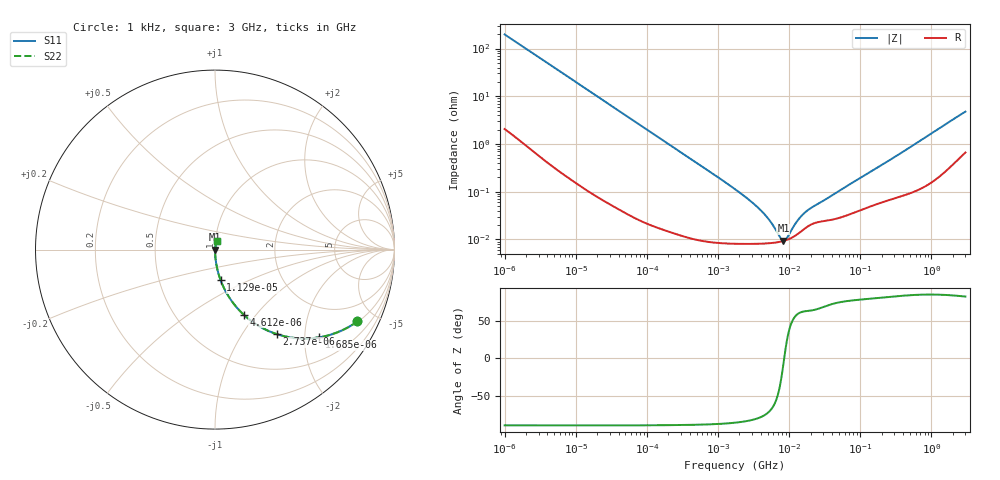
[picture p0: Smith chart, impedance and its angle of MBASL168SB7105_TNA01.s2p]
! MBASL168SB7105_TNA01  S-PARAMETER MODEL  ( Standard Model )
! Model Generated by TAIYO YUDEN Corporation (http://www.ty-top.com)
! Version 1.0
! TAIYO YUDEN Control No. 220601
! Copyright(c) 2012 TAIYO YUDEN CO.,LTD. All Rights Reserved.
! Product Description (link to TY-COMPAS)
! https://ds.yuden.co.jp/TYCOMPAS/or/detail?pn=MBASL168SB7105KTNA01&u=M
! Products Name : Multilayer Ceramic Capacitors
! Characteristics :
!  Capacitance : 1 [uF] , Rated Voltage : 10 [V] , TCC : X7R
!  Case Size : 1.6 x 0.8 / 0.063 x 0.031 [mm/inch] , Thickness : 0.8 / 0.031 [mm/inch]
!  (Conditions: Temperature = 25 [degC] , DC Bias Voltage = 0 [V])
! External Node Assignments :
!  1  o---| |---o  2
! GND o---------o GND
! Frequency Range : 1kHz  -  3GHz  [ 401 STEP ]
# MHZ S RI R 50
! Freq[MHz].  S11 Real  S11 Imag  S21 Real  S21 Imag  S12 Real  S12 Imag  S22 Real  S22 Imag
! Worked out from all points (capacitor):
!   401 points, 1 kHz to 3 GHz, reference 50 ohm
!   read as one part in series: C = 805 nF near 1.077 kHz
!   lowest |Z| = 9.36 mohm at 8.292 MHz (marker M1)
!   series resonance near 8.517 MHz, so ESL is about 430 pH
!   S11 on the Smith chart (normalised r, x): 1 kHz: 1.04, -3.94; 1.685 kHz: 1.02, -2.35; 2.737 kHz: 1.01, -1.45; 4.612 kHz: 1.01, -0.86; 11.29 kHz: 1.00, -0.35; 3 GHz: 1.01, +0.09
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0.001  0.7929 -0.4  0.2071 0.4  0.2071 0.4  0.7929 -0.4
0.001685  0.579 -0.4889  0.421 0.4889  0.421 0.4889  0.579 -0.4889
0.002737  0.3461 -0.4714  0.6539 0.4714  0.6539 0.4714  0.3461 -0.4714
0.004612  0.159 -0.3617  0.841 0.3617  0.841 0.3617  0.159 -0.3617
0.006951  0.0778 -0.264  0.9222 0.264  0.9222 0.264  0.0778 -0.264
0.011286  0.0316 -0.1712  0.9684 0.1712  0.9684 0.1712  0.0316 -0.1712
0.01216  0.0275 -0.1597  0.9725 0.1597  0.9725 0.1597  0.0275 -0.1597
0.033275  0.00412 -0.06  0.9959 0.06  0.9959 0.06  0.00412 -0.06
0.147855  0.000358 -0.0137  0.9996 0.0137  0.9996 0.0137  0.000358 -0.0137
1.732051  8.23e-05 -0.00113  0.9999 0.00113  0.9999 0.00113  8.23e-05 -0.00113
2.812335  8.1e-05 -0.000647  0.9999 0.000647  0.9999 0.000647  8.1e-05 -0.000647
4.083148  8.17e-05 -0.000386  0.9999 0.000386  0.9999 0.000386  8.17e-05 -0.000386
5.502215  8.39e-05 -0.000217  0.9999 0.000217  0.9999 0.000217  8.39e-05 -0.000217
7.414467  8.92e-05 -6.73e-05  0.9999 6.73e-05  0.9999 6.73e-05  8.92e-05 -6.73e-05
8.291982  9.27e-05 -1.29e-05  0.9999 1.29e-05  0.9999 1.29e-05  9.27e-05 -1.29e-05
8.933959  9.58e-05 2.33e-05  0.9999 -2.33e-05  0.9999 -2.33e-05  9.58e-05 2.33e-05
9.625639  9.98e-05 5.96e-05  0.9999 -5.96e-05  0.9999 -5.96e-05  9.98e-05 5.96e-05
12.03889  0.000118 0.00017  0.9999 -0.00017  0.9999 -0.00017  0.000118 0.00017
14.50609  0.000145 0.000261  0.9999 -0.000261  0.9999 -0.000261  0.000145 0.000261
21.06097  0.000211 0.000424  0.9998 -0.000424  0.9998 -0.000424  0.000211 0.000424
256.0921  0.00069 0.0045  0.9993 -0.0045  0.9993 -0.0045  0.00069 0.0045
3000  0.00876 0.0464  0.9912 -0.0464  0.9912 -0.0464  0.00876 0.0464
